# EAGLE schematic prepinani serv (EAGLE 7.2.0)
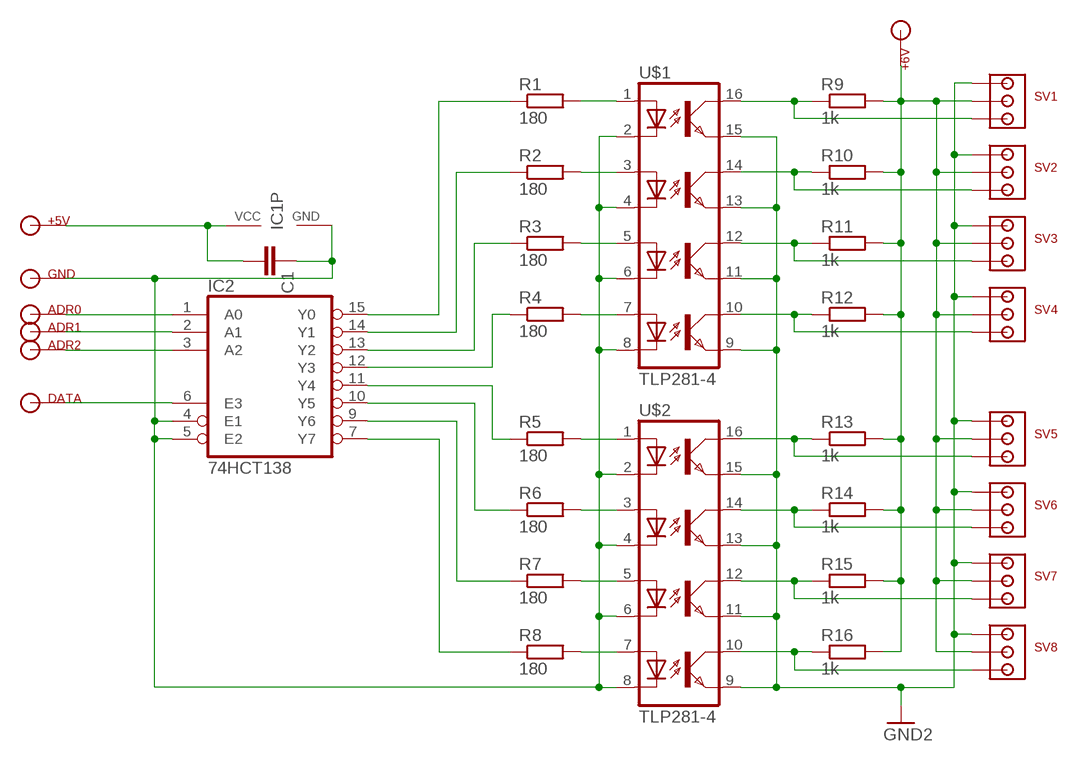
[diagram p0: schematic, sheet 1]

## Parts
C1  C-EUC1206  [C1206]
IC1  74AC138D  [SO16]
IC2  74HCT138  74HCT138D  [SO16]
R1  180  R-EU_R1206  [R1206]
R2  180  R-EU_R1206  [R1206]
R3  180  R-EU_R1206  [R1206]
R4  180  R-EU_R1206  [R1206]
R5  180  R-EU_R1206  [R1206]
R6  180  R-EU_R1206  [R1206]
R7  180  R-EU_R1206  [R1206]
R8  180  R-EU_R1206  [R1206]
R9  1k  R-EU_R1206  [R1206]
R10  1k  R-EU_R1206  [R1206]
R11  1k  R-EU_R1206  [R1206]
R12  1k  R-EU_R1206  [R1206]
R13  1k  R-EU_R1206  [R1206]
R14  1k  R-EU_R1206  [R1206]
R15  1k  R-EU_R1206  [R1206]
R16  1k  R-EU_R1206  [R1206]
U$1  TLP281-4  [MINI-FLAT-16]
U$2  TLP281-4  [MINI-FLAT-16]
U$4  ADR0  MOJE_1  [MOJE_1]
U$5  ADR1  MOJE_1  [MOJE_1]
U$6  SV1  MOJE_3  [MOJE_3]
U$7  SV2  MOJE_3  [MOJE_3]
U$8  SV3  MOJE_3  [MOJE_3]
U$9  SV4  MOJE_3  [MOJE_3]
U$10  SV5  MOJE_3  [MOJE_3]
U$11  SV6  MOJE_3  [MOJE_3]
U$12  SV7  MOJE_3  [MOJE_3]
U$13  SV8  MOJE_3  [MOJE_3]
U$14  ADR2  MOJE_1  [MOJE_1]
U$15  GND  MOJE_1  [MOJE_1]
U$16  +5V  MOJE_1  [MOJE_1]
U$17  +6V  MOJE_1  [MOJE_1]
U$18  DATA  MOJE_1  [MOJE_1]

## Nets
GND: U$1.9(EMIT3) U$1.11(EMIT2) U$1.13(EMIT1) U$1.15(EMIT) U$2.9(EMIT3) U$2.11(EMIT2) U$2.13(EMIT1) U$2.15(EMIT) U$6.P$1 U$7.P$1 U$8.P$1 U$9.P$1 U$10.P$1 U$11.P$1 U$12.P$1 U$13.P$1 ; supply symbol labelled GND2
N$1: R9.1 U$1.16(COL) U$6.P$3
N$2: R10.1 U$1.14(COL1) U$7.P$3
N$3: R11.1 U$1.12(COL2) U$8.P$3
N$4: R12.1 U$1.10(COL3) U$9.P$3
N$5: R13.1 U$2.16(COL) U$10.P$3
N$6: R14.1 U$2.14(COL1) U$11.P$3
N$7: R15.1 U$2.12(COL2) U$12.P$3
N$8: R16.1 U$2.10(COL3) U$13.P$3
N$12: R1.2 U$1.1(A)
N$13: R2.2 U$1.3(A1)
N$14: R3.2 U$1.5(A2)
N$15: R4.2 U$1.7(A3)
N$16: R5.2 U$2.1(A)
N$17: R6.2 U$2.3(A1)
N$18: R7.2 U$2.5(A2)
N$19: R8.2 U$2.7(A3)
N$20 [GND1]: C1.1 IC1.8(GND) IC2.4(E1) IC2.5(E2) U$1.2(C) U$1.4(C1) U$1.6(C2) U$1.8(C3) U$2.2(C) U$2.4(C1) U$2.6(C2) U$2.8(C3) U$15.P$1
N$22: IC2.12(Y3) R4.1
N$23: IC2.13(Y2) R3.1
N$24: IC2.14(Y1) R2.1
N$25: IC2.15(Y0) R1.1
N$26: IC2.11(Y4) R5.1
N$27: IC2.10(Y5) R6.1
N$28: IC2.9(Y6) R7.1
N$29: IC2.7(Y7) R8.1
N$30: IC2.1(A0) U$4.P$1
N$31: IC2.2(A1) U$5.P$1
N$32: IC2.3(A2) U$14.P$1
N$34: IC2.6(E3) U$18.P$1
N$43 [VCC2]: R9.2 R10.2 R11.2 R12.2 R13.2 R14.2 R15.2 R16.2 U$6.P$2 U$7.P$2 U$8.P$2 U$9.P$2 U$10.P$2 U$11.P$2 U$12.P$2 U$13.P$2 U$17.P$1
N$65: C1.2 IC1.16(VCC) U$16.P$1
Unconnected: IC1.1(A0) IC1.2(A1) IC1.3(A2) IC1.4(E1) IC1.5(E2) IC1.6(E3) IC1.7(Y7) IC1.9(Y6) IC1.10(Y5) IC1.11(Y4) IC1.12(Y3) IC1.13(Y2) IC1.14(Y1) IC1.15(Y0)

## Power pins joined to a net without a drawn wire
GND: IC2.8(GND)
VCC: IC2.16(VCC)

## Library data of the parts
C1 = rcl:C-EU: CAPACITOR, European symbol
IC1 IC2 = 74xx-eu:74*138: 3-line to 8-line DECODER/DEMULTIPLEXER
R1-R16 = rcl:R-EU_: RESISTOR, European symbol
U$1 U$2 = optocoupler:TLP281-4
U$4 U$5 U$14-U$18 = con-lstb:MOJE_1
U$6-U$13 = con-lstb:MOJE_3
